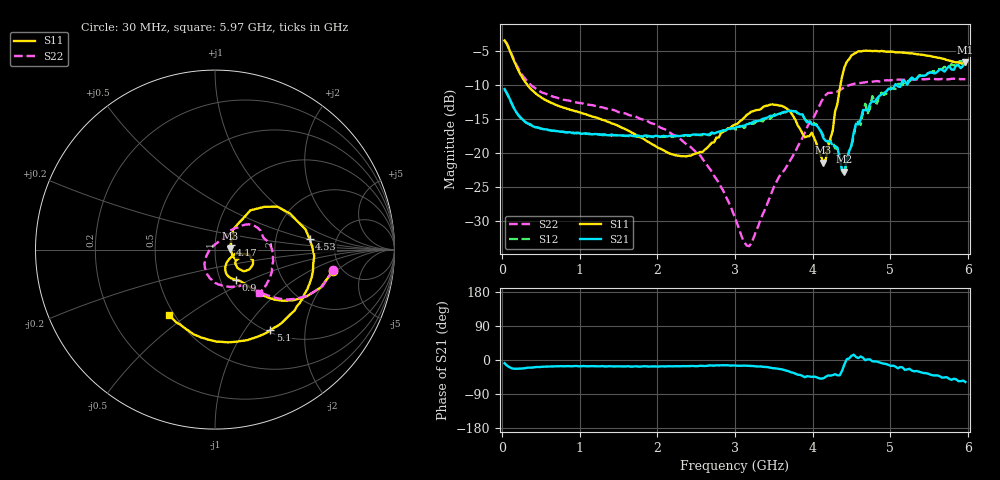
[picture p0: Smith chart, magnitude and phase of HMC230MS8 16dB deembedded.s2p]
!Hittite Microwave Corporation
!12 Elizabeth Drive
!Chelmsford, MA 01824
!Tel: 978-250-3343
!Fax: 978-250-3373
!Device: HMC230MS8, 0.75-2 GHz GaAs IC 3-bit Digital Attenuator in 8 lead plastic surface mount Mini Small Outline Package
!Misc: Room Temp Vdd = 5V , 16dB State.
# GHZ S DB R 50.0
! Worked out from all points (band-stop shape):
!   199 points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, 30 MHz to 5.97 GHz, reference 50 ohm
!   highest |S21| = -6.72 dB at 5.97 GHz (marker M1); lowest = -22.7 dB at 4.41 GHz (marker M2)
!   |S21| within 3 dB of the highest: 5.149 GHz to 5.204 GHz (55 MHz wide, 1.06 % of centre); 5.232 GHz to end of sweep
!   lowest |S11| = -21.4 dB at 4.14 GHz (marker M3), VSWR 1.19, Z = 59.3 + j0.559 ohm
!   |S11| at or under -10 dB: 321.1 MHz to 4.36 GHz (4.039 GHz wide, 173 % of centre)
!   |S22| runs from -33.6 to -3.5 dB; largest |S21 - S12| = 0.064
!   S11 on the Smith chart (normalised r, x): 30 MHz: 4.16, -1.81; 900 MHz: 1.19, -0.42; 4.17 GHz: 1.19, +0.06; 4.53 GHz: 3.16, +0.53; 5.1 GHz: 1.03, -1.32; 5.97 GHz: 0.47, -0.43
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0.03  -3.53 -10.5  -10.64 -8.5  -10.72 -8.2  -3.53 -10.0
0.12  -5.66 -32.8  -12.67 -21.9  -12.77 -21.4  -5.52 -31.2
0.27  -9.17 -44.7  -15.19 -22.2  -15.18 -21.7  -8.78 -42.4
0.9  -13.75 -55.2  -17.07 -16.6  -16.96 -16.4  -12.46 -58.8
1.02  -14.14 -57.5  -17.20 -16.3  -17.10 -16.7  -12.69 -63.3
2.04  -19.37 -56.7  -17.63 -16.7  -17.61 -16.8  -16.28 -103.0
2.55  -19.84 -22.5  -17.32 -15.3  -17.39 -15.4  -20.34 -127.1
3  -15.82 -9.0  -16.30 -14.5  -16.54 -15.7  -29.51 -168.5
3.21  -13.94 -10.8  -15.60 -15.3  -15.69 -15.7  -33.27 117.3
3.6  -13.08 -28.6  -14.15 -24.5  -14.11 -23.1  -22.88 54.9
3.99  -17.02 -21.7  -15.78 -44.5  -15.79 -42.5  -15.03 43.9
4.14  -21.39 3.1  -17.83 -48.2  -17.51 -47.4  -11.90 32.1
4.17  -20.88 16.6  -18.22 -44.1  -17.97 -45.4  -11.50 27.3
4.32  -12.82 47.9  -19.20 -40.4  -19.33 -38.3  -11.00 12.3
4.41  -7.49 34.5  -22.73 -11.8  -23.07 -11.4  -10.35 7.4
4.53  -5.51 6.5  -17.01 14.0  -17.64 14.7  -9.89 -2.1
4.68  -5.03 -16.1  -13.70 -0.6  -12.78 -0.0  -9.64 -10.6
4.71  -5.04 -19.6  -13.81 1.8  -14.18 -3.5  -9.60 -11.7
4.98  -5.16 -45.6  -10.59 -13.0  -10.87 -10.2  -9.37 -22.4
5.1  -5.27 -55.6  -10.25 -22.0  -9.90 -15.6  -9.25 -26.4
5.52  -5.81 -89.2  -8.20 -38.8  -8.16 -34.6  -9.13 -37.2
5.97  -7.02 -125.1  -6.72 -58.1  -6.60 -52.0  -9.20 -44.5
